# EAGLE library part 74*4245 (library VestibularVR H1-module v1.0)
Octal BUS TRANSCEIVER, 3-state
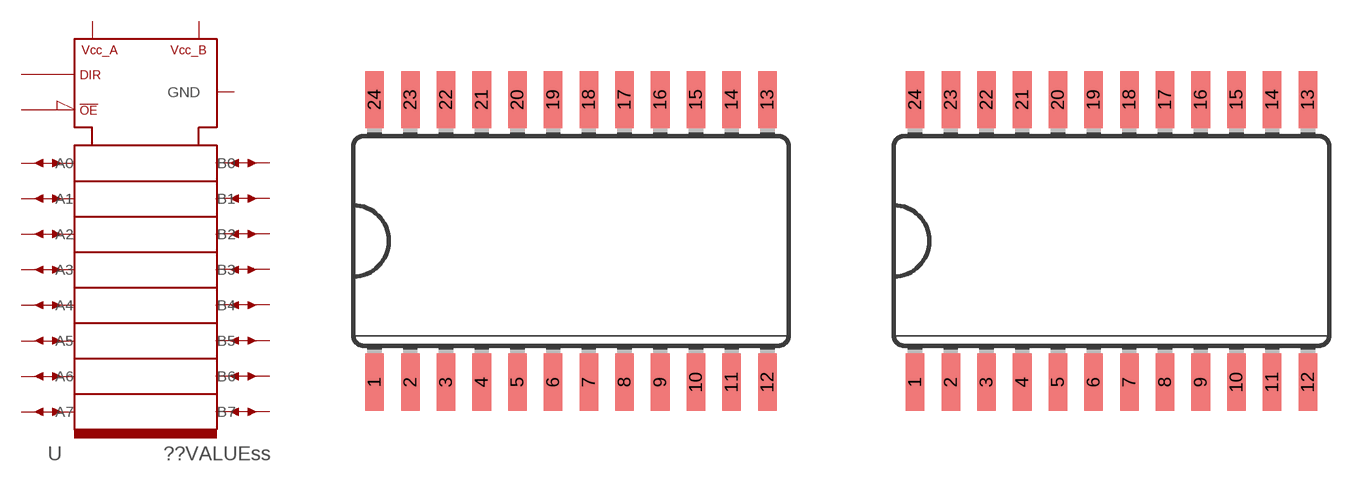
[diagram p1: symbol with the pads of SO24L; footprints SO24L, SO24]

Designator prefix U

## 744245TECH2  [SO24L]
1  VCC_A  in
2  DIR  in
3  A0
4  A1
5  A2
6  A3
7  A4
8  A5
9  A6
10  A7
11  GND
12  GND
13  GND
14  B7
15  B6
16  B5
17  B4
18  B3
19  B2
20  B1
21  B0
22  OE  in
23  VCC_B  in
24  VCC_B  in

## 744245, 74TECH24245  [SO24]
Pads as for SO24L

## Footprint SO24L (pad centres in mm)
24-Lead (300-Mil) SOIC S13 Source: www.cypress.com .. CY7C6301XX.pdf
smd 0.66 x 2.032: 1 -6.985,-5.029; 2 -5.715,-5.029; 3 -4.445,-5.029; 4 -3.175,-5.029; 5 -1.905,-5.029; 6 -0.635,-5.029; 7 0.635,-5.029; 8 1.905,-5.029; 9 3.175,-5.029; 10 4.445,-5.029; 11 5.715,-5.029; 12 6.985,-5.029; 13 6.985,5.029; 14 5.715,5.029; 15 4.445,5.029; 16 3.175,5.029; 17 1.905,5.029; 18 0.635,5.029; 19 -0.635,5.029; 20 -1.905,5.029; 21 -3.175,5.029; 22 -4.445,5.029; 23 -5.715,5.029; 24 -6.985,5.029

## Footprint SO24 (pad centres in mm)
24-Lead (300-Mil) SOIC S13 Source: www.cypress.com .. CY7C6301XX.pdf
smd 0.66 x 2.032: 1 -6.985,-5.029; 2 -5.715,-5.029; 3 -4.445,-5.029; 4 -3.175,-5.029; 5 -1.905,-5.029; 6 -0.635,-5.029; 7 0.635,-5.029; 8 1.905,-5.029; 9 3.175,-5.029; 10 4.445,-5.029; 11 5.715,-5.029; 12 6.985,-5.029; 13 6.985,5.029; 14 5.715,5.029; 15 4.445,5.029; 16 3.175,5.029; 17 1.905,5.029; 18 0.635,5.029; 19 -0.635,5.029; 20 -1.905,5.029; 21 -3.175,5.029; 22 -4.445,5.029; 23 -5.715,5.029; 24 -6.985,5.029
